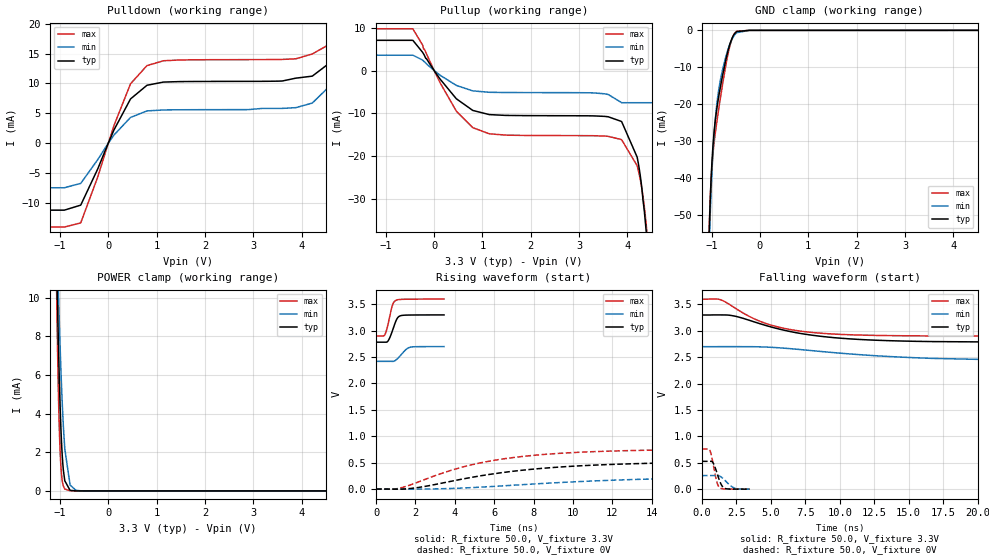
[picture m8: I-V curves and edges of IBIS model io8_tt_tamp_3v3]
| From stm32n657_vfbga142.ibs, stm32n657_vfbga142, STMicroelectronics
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[Model]   io8_tt_tamp_3v3
Model_type I/O
Polarity   Non-Inverting
Enable   Active-Low
| CAP_THRESHOLD on pad IOTT is "UDTCAPC" :
| Rising=30.0% of vddiov33m   Falling=70.0% of vddiov33m
| C_comp min and max val. don't necessarily correlate with the min and max pvt
| but are the smallest and greatest pad capacitance found.
| var   typ   min   max
C_comp   1.36103pF  1.35590pF  1.37594pF
|C_comp_pullup   660.49000fF  643.07500fF  686.64000fF
|C_comp_pulldown   700.53500fF  712.82730fF  689.29500fF
Vinl = 810.0mV
Vinh = 2.52V
Vmeas = 1.65V   | Reference voltage for timing measurements
Cref  = 50.0pF   | Timing specification test load capacitance value
Rref  = 100.0MOhm   | Timing specification test load resistance value
Vref  = 1.65V   | Timing specification test load voltage
[Model Spec]
| TIME_THRESHOLD on pin ZIV08SW is "CMOS" :
| Rising=50.0% of vddv08sw   Falling=50.0% of vddv08sw
Vinl 1.08570V 868.70000mV 1.21270V
Vinh 1.55630V 1.26230V 1.70930V
| variable   typ   min   max
[Temperature Range] 25.0 125.0 -40.0
| variable   typ   min   max
[Voltage Range] 3.3V 2.7V 3.6V
| variable   typ   min   max
[POWER Clamp Reference] 3.3V 2.7V 3.6V
| variable   typ   min   max
[GND Clamp Reference] 0V 0V 0V
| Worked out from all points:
|   slope of the pulldown table from 0 to 0.495 V, typ, clamps not added: 64.8 ohm
|   slope of the pullup table from 0 to 0.495 V, typ, clamps not added: 71.9 ohm
|   GND clamp passes 1 mA (typ) near -0.53 V on its own axis
|   POWER clamp passes 1 mA (typ) near -0.93 V on its own axis
|   rising waveform, R_fixture 50.0, V_fixture 3.3V: 20-80 % time 305ps typ, 418ps min, 260ps max; typ from 2.78 V to 3.3 V
|   falling waveform, R_fixture 50.0, V_fixture 3.3V: 20-80 % time 5.52ns typ, 9.98ns min, 3.85ns max; typ from 3.3 V to 2.78 V
|   rising waveform, R_fixture 50.0, V_fixture 0V: 20-80 % time 6.28ns typ, 9.89ns min, 4.94ns max; typ from 0 V to 0.528 V
|   falling waveform, R_fixture 50.0, V_fixture 0V: 20-80 % time 428ps typ, 636ps min, 354ps max; typ from 0.528 V to 0.001 V
[POWER Clamp]
-3.3V     1.38A      323.1mA    2.043A
-1.07V    12.25mA    13.83mA    10.54mA
-1.06V    10.95mA    12.87mA    8.878mA
-1.05V    9.713mA    11.93mA    7.364mA
-1.03V    7.451mA    10.15mA    4.822mA
-1V       4.658mA    7.711mA    2.251mA
-980mV    3.232mA    6.265mA    1.26mA
-950mV    1.731mA    4.404mA    492.1uA
-900mV    524.1uA    2.175mA    97.66uA
-790mV    30.71uA    308.1uA    7.362uA
-670mV    2.544uA    30.85uA    4.15uA
6.6V      0A         0A         0A
[GND Clamp]
-3.3V     -3.81A     -3.793A    -3.82A
-1.05V    -55.06mA   -58.88mA   -53.92mA
-1.04V    -50.66mA   -54.44mA   -49.72mA
-1.03V    -46.76mA   -50.42mA   -46.13mA
-1V       -37.5mA    -40.39mA   -38.26mA
-970mV    -31mA      -32.73mA   -33.22mA
-920mV    -24.01mA   -23.65mA   -27.5mA
-860mV    -18.53mA   -16.79mA   -21.95mA
-770mV    -12.04mA   -10.49mA   -14.37mA
-640mV    -4.528mA   -4.381mA   -5.198mA
-480mV    -339.7uA   -626.6uA   -256.2uA
6.6V      277.9nA    5.113uA    319.8nA
| variable   typ   min   max
[Pullup Reference] 3.3V 2.7V 3.6V
| variable   typ   min   max
[Pulldown Reference] 0V 0V 0V
[Pullup]
-3.3V     7.045mA    3.581mA    9.738mA
-440mV    7.045mA    3.581mA    9.729mA
460mV     -6.603mA   -3.484mA   -9.498mA
800mV     -9.321mA   -4.753mA   -13.34mA
1.48V     -10.48mA   -5.137mA   -15.08mA
3.3V      -10.59mA   -5.231mA   -15.22mA
3.87V     -11.87mA   -7.44mA    -16.11mA
4.2V      -20.22mA   -7.52mA    -22.23mA
4.3V      -27.8mA    -7.52mA    -27.83mA
4.38V     -36.68mA   -7.52mA    -35.12mA
4.39V     -38mA      -7.52mA    -36.28mA
6.6V      -45.55mA   -7.52mA    -114mA
[Pulldown]
-3.3V     -11.22mA   -7.47mA    -14.05mA
-910mV    -11.22mA   -7.47mA    -14.05mA
-570mV    -10.38mA   -6.74mA    -13.35mA
120mV     2.252mA    1.384mA    2.997mA
460mV     7.403mA    4.305mA    9.944mA
800mV     9.691mA    5.396mA    12.98mA
3.6V      10.41mA    5.819mA    14.02mA
4.22V     11.22mA    6.711mA    14.93mA
4.56V     13.31mA    9.4mA      16.48mA
4.9V      20.4mA     17.95mA    22.54mA
5.24V     41.73mA    41.86mA    41.61mA
6.6V      249.9mA    252.7mA    243mA
[Ramp]
dV/dt_r 316.76783mV/6.27755ns 154.94103mV/9.7568ns 455.99382mV/4.93807ns
dV/dt_f 310.40072mV/5.51352ns 168.27652mV/9.82155ns 419.59266mV/3.84848ns
R_load = 50.0
| Removed startup time: 0s 0s 0s  .
| Removed end time: 3.45ns.
[Rising Waveform]
R_fixture   = 50.0
V_fixture   = 3.3V
V_fixture_min = 2.7V
V_fixture_max = 3.6V
0s        2.783V     2.42V      2.901V
400ps     2.783V     2.42V      2.902V
450ps     2.783V     2.42V      2.927V
600ps     2.802V     2.42V      3.112V
800ps     2.968V     2.42V      3.446V
900ps     3.076V     2.421V     3.54V
1ns       3.179V     2.443V     3.574V
1.2ns     3.278V     2.515V     3.592V
1.7ns     3.297V     2.684V     3.597V
3.45ns    3.299V     2.699V     3.599V
| Removed startup time: 0s 0s 0s  .
| Removed end time: 69.9ns.
[Falling Waveform]
R_fixture   = 50.0
V_fixture   = 3.3V
V_fixture_min = 2.7V
V_fixture_max = 3.6V
0s        3.3V       2.7V       3.6V
1.4ns     3.301V     2.701V     3.584V
2.4ns     3.278V     2.701V     3.432V
3.8ns     3.169V     2.699V     3.227V
5.5ns     3.041V     2.68V      3.074V
7.4ns     2.94V      2.639V     2.986V
10.3ns    2.856V     2.571V     2.93V
15.6ns    2.801V     2.489V     2.905V
23.3ns    2.785V     2.441V     2.901V
69.9ns    2.783V     2.42V      2.901V
| Removed startup time: 0s 0s 0s  .
| Removed end time: 69.9ns.
[Rising Waveform]
R_fixture   = 50.0
V_fixture   = 0V
V_fixture_min = 0V
V_fixture_max = 0V
0s        940.4nV    5.057uV    1.136uV
1.2ns     -734.7uV   -700.6uV   18.51mV
2.3ns     39.36mV    893.5nV    156.5mV
4.1ns     169.1mV    15.36mV    387mV
6.1ns     296mV      53.44mV    550.7mV
8.4ns     391.3mV    104.8mV    652.1mV
11.8ns    464.6mV    164.8mV    718.5mV
15.6ns    500.3mV    205.2mV    745.3mV
23.3ns    522.5mV    240.6mV    758.1mV
69.9ns    527.9mV    258.2mV    760mV
| Removed startup time: 0s 0s 0s  .
| Removed end time: 3.45ns.
[Falling Waveform]
R_fixture   = 50.0
V_fixture   = 0V
V_fixture_min = 0V
V_fixture_max = 0V
0s        527.9mV    258.3mV    760mV
550ps     527.9mV    258.3mV    750.8mV
700ps     528.6mV    258.3mV    623.6mV
850ps     477.5mV    258.3mV    427.8mV
1.1ns     299.5mV    258.4mV    120.6mV
1.3ns     146.4mV    247.1mV    24.93mV
1.5ns     47.57mV    209mV      7.259mV
1.7ns     12.1mV     159.3mV    3.614mV
2.35ns    1.751mV    23.86mV    1.365mV
3.45ns    620.5uV    844.3uV    519.4uV
